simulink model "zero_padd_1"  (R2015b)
settings: Solver=ode45  StartTime=0.0  StopTime=10.0  RelTol=1e-3
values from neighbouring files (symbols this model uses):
  fsig1 = 100.5    [leakage_3.m]    (also in leakage_4.m; zero_padd1.m = 100; zero_padd2.m = 100; zero_padd3.m = 100)
  fsig2 = 150.3    [leakage_3.m]    (also in leakage_4.m; zero_padd1.m = ',num2str(fsig2),' Hz und N = ',     num2str(N),' bzw. nfft ; zero_padd2.m = ',num2str(fsig2),' Hz und N = ',     num2str(N),' bzw. nfft ; zero_padd3.m = ',num2str(fsig2),' Hz und N = ',     num2str(N),' bzw. nfft )
  N = 4*1024    (= 4096)    [ad_test_12.m]    (also in ad_test_2.m; ad_test_3.m; DA_wandler_spektr_1.m = 1000; DA_wandler_spektr_2.m = 1024)
  nfft = 2^p2    [DA_wandler_spektr_1.m]    (also in DA_wandler_spektr_2.m; PSD_korrelation_1.m = 2^(nextpow2(2*lag_max)); welch_1.m = 256; zero_padd1.m = ',num2str(nfft),')
  Ts = 1/fs    (= 0.00025)    [abtast_rate_1.m]    (also in ad_test_12.m = 0.0009765625; ad_test_2.m = 0.00048828125; ad_test_3.m = 0.00048828125; DA_wandler_spektr_1.m = 0.01)
undefined symbols (not defined in the file or in its folder): get
libraries: dspspect3 x1, dspsnks4 x1, dspsigops x1

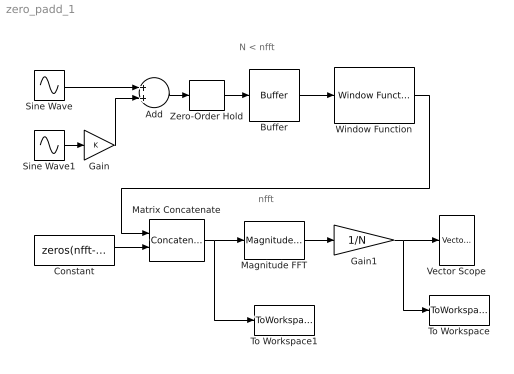
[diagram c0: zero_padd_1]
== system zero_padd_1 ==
  note: N < nfft
  note: nfft
  Add : Sum
  Buffer : Buffer  N=N  TreatMby1Signals=One channel
  Constant : Constant  Value=zeros(nfft-N, 1)
  Gain : Gain
  Gain1 : Gain  Gain=1/N
  Magnitude FFT : dspspect3/Magnitude FFT  mag_or_magsq=Magnitude  FFTImplementation=Auto  fftLenInherit=off  fftsize=nfft  WrapInput=on
  Matrix Concatenate : Concatenate  Mode=Multidimensional array
  Sine Wave : Sin  Frequency=2*pi*fsig1  SampleTime=0
  Sine Wave1 : Sin  Frequency=2*pi*fsig2  SampleTime=0
  To Workspace : ToWorkspace  VariableName=y  SaveFormat=Structure  SampleTime=-1
  To Workspace1 : ToWorkspace  VariableName=y1  SaveFormat=Structure  SampleTime=-1
  Vector Scope : dspsnks4/Vector Scope  ScopeProperties=on  Domain=Frequency  HorizSpan=1  DisplayProperties=off  AxisGrid=on  Memory=off  FrameNumber=on  AxisLegend=off  AxisZoom=off  OpenScopeAtSimStart=on  OpenScopeImmediately=off  FigPos=get(0,'defaultfigureposition')  AxisProperties=off  XUnits=Hertz  XRange=[0...Fs]  InheritXIncr=off  XIncr=1/1000  XLabel=Time  XLimit=User-defined  XMin=2.1333  XMax=1000.5333  XStart=0  YUnits=Magnitude  YLabel=Amplitude  LineProperties=off  XAxisParamsVer=6.9
  Window Function : dspsigops/Window Function  winmode=Apply window to input  wintype=Boxcar  sampmode=Continuous  samptime=1  N=64  Rs=50  beta=10  winsamp=Symmetric  UserWindow=hamming  OptParams=off  UserParams={'symmetric'}  dataType=double  isSigned=on  wordLen=16  udDataType=sfix(16)  fracBitsMode=Best precision  numFracBits=15  roundingMode=Floor  overflowMode=off  numSidelobes=4  sidelobeLevel=-30
  Zero-Order Hold : ZeroOrderHold  SampleTime=Ts
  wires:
  Sine Wave1/1 -> Gain/1
  Sine Wave/1 -> Add/1
  Gain/1 -> Add/2
  Add/1 -> Zero-Order Hold/1
  Zero-Order Hold/1 -> Buffer/1
  Magnitude FFT/1 -> Gain1/1
  Gain1/1 -> To Workspace/1, Vector Scope/1
  Buffer/1 -> Window Function/1
  Matrix Concatenate/1 -> To Workspace1/1, Magnitude FFT/1
  Constant/1 -> Matrix Concatenate/2
  Window Function/1 -> Matrix Concatenate/1
